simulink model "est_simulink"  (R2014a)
settings: Solver=ode45  StartTime=0.0  StopTime=20  RelTol=1e-3
StartFcn:
  | clear all
libraries: simulink x1

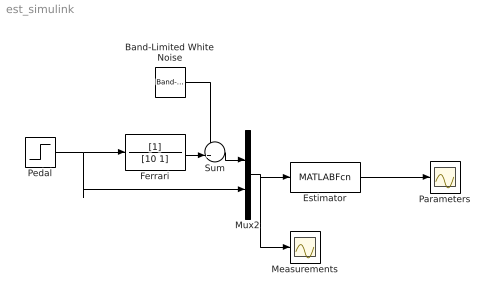
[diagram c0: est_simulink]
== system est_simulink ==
  Band-Limited White Noise : simulink/Sources/Band-Limited White Noise  Cov=[0.1]  Ts=1  seed=[23341]
  Estimator : MATLABFcn  MATLABFcn=est_apm  SampleTime=1
  Ferrari : TransferFcn  Denominator=[10 1]
  Measurements : Scope
  Mux2 : Mux  Inputs=2
  Parameters : Scope
  Pedal : Step  Time=3.01  After=100  SampleTime=0
  Sum : Sum  Inputs=++|
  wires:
  Mux2/1 -> Measurements/1, Estimator/1
  Estimator/1 -> Parameters/1
  Pedal/1 -> Mux2/2, Ferrari/1
  Ferrari/1 -> Sum/2
  Sum/1 -> Mux2/1
  Band-Limited White Noise/1 -> Sum/1
